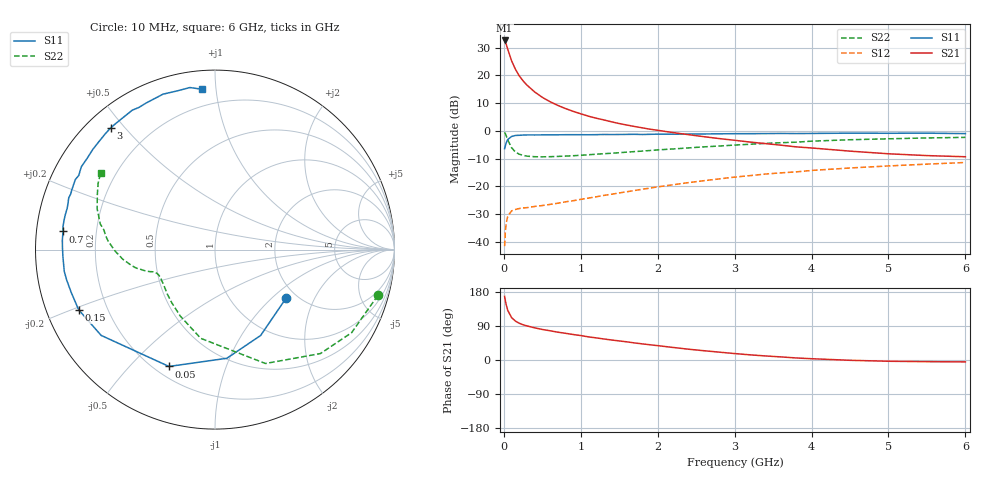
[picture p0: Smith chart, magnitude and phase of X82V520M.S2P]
! SIEMENS Small Signal Semiconductors
! BFP136W
! Si NPN RF Bipolar Junction Transistor in SOT343
! VCE = 2.5 V  IC = 20 mA
! Common Emitter S-Parameters:  September  1994
# GHz  S  MA  R  50
!  f  S11  S21  S12  S22
! GHz  MAG  ANG  MAG  ANG  MAG  ANG  MAG  ANG
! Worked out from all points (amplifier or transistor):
!   40 points, 10 MHz to 6 GHz, reference 50 ohm
!   highest |S21| = 32.6 dB at 10 MHz (marker M1)
!   |S21| within 3 dB of that: start of sweep to 48.81 MHz
!   unconditionally stable (mu >= 1): 853.9 MHz to 2.766 GHz
!   at 200 MHz: K = 0.33, MSG = 23.9 dB, |S12| = -27.9 dB
!   at 1.5 GHz: K = 1.16, MAG = 10.1 dB, |S12| = -22.3 dB
!   at 6 GHz: K = 0.99, MSG = 1.0 dB, |S12| = -11.4 dB
!   S11 on the Smith chart (normalised r, x): 10 MHz: 1.76, -1.24; 50 MHz: 0.25, -0.65; 150 MHz: 0.10, -0.21; 700 MHz: 0.08, +0.06; 3 GHz: 0.07, +0.46; 6 GHz: 0.10, +0.92
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0.01  0.4797 -34.2  42.73 167.8  0.0084 76.4  0.9426 -15.7
0.02  0.5418 -62.0  39.89 156.1  0.0154 68.8  0.8908 -31.3
0.03  0.6092 -83.8  36.92 146.5  0.0215 58.4  0.8249 -44.6
0.05  0.6997 -111.5  29.87 131.3  0.0288 44.5  0.6942 -66.1
0.1  0.7943 -143.0  18.51 112.1  0.0363 30.3  0.5008 -99.1
0.15  0.8303 -156.2  12.98 102.7  0.0384 25.7  0.418 -117.5
0.2  0.8357 -163.3  9.864 97.0  0.0401 24.3  0.3818 -129.1
0.25  0.8436 -168.4  7.995 93.0  0.041 24.0  0.3635 -136.9
0.3  0.8486 -171.8  6.707 90.0  0.0415 24.6  0.3518 -142.3
0.4  0.8481 -177.2  5.056 84.9  0.0437 26.8  0.3437 -149.2
0.5  0.8501 179.1  4.038 80.6  0.0453 29.6  0.3418 -153.4
0.6  0.8521 176.4  3.367 77.2  0.0475 32.4  0.3441 -155.7
0.7  0.8528 173.2  2.896 73.5  0.0499 35.3  0.3477 -157.2
0.9  0.8567 169.1  2.26 67.3  0.0554 39.8  0.3579 -159.5
1.1  0.8552 164.4  1.846 61.0  0.0618 43.9  0.3728 -160.7
1.5  0.8641 157.5  1.361 50.3  0.0764 49.5  0.406 -163.1
2.2  0.8751 144.6  0.935 33.1  0.1074 52.0  0.474 -169.3
3  0.8934 130.5  0.679 17.0  0.1474 48.7  0.557 -179.2
3.2  0.8946 127.1  0.631 13.6  0.1569 47.4  0.5762 178.1
4.5  0.9131 108.5  0.433 -0.8  0.2153 36.0  0.6948 160.9
5.5  0.9137 98.8  0.36 -4.4  0.2527 27.6  0.7485 150.5
6  0.8958 94.5  0.343 -5.0  0.2706 22.9  0.767 146.2
